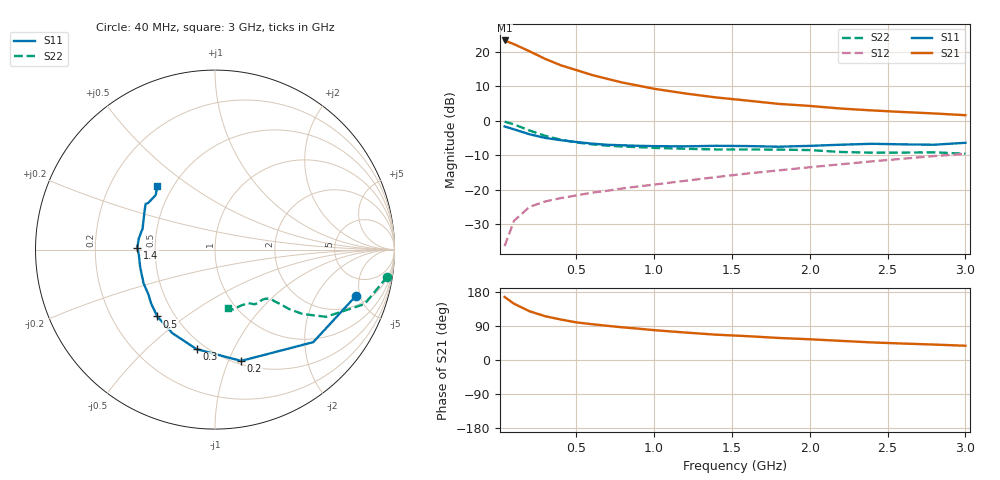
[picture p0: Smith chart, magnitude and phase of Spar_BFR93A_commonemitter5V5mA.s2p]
! Filename:  BFR93AA.S2P  Version:  2.0
! NXP part #: BFR93A  Date: May 1990
! Bias condition: Vce=5V, Ic=5mA
#  MHz  S  MA  R  50
! Freq  S11  S21  S12  S22  !GUM [dB]
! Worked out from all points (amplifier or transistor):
!   21 points, 40 MHz to 3 GHz, reference 50 ohm
!   highest |S21| = 23.4 dB at 40 MHz (marker M1)
!   |S21| within 3 dB of that: start of sweep to 192.8 MHz
!   unconditionally stable (mu >= 1): 1.032 GHz to 2.386 GHz
!   at 300 MHz: K = 0.48, MSG = 20.8 dB, |S12| = -23.5 dB
!   at 1 GHz: K = 0.99, MSG = 13.9 dB, |S12| = -18.6 dB
!   at 3 GHz: K = 0.95, MSG = 5.6 dB, |S12| = -9.6 dB
!   S11 on the Smith chart (normalised r, x): 40 MHz: 2.83, -4.60; 200 MHz: 0.53, -1.11; 300 MHz: 0.45, -0.73; 500 MHz: 0.40, -0.40; 1.4 GHz: 0.40, +0.01; 3 GHz: 0.41, +0.38
40  0.827 -18.1  14.76 166.3  0.015 78.6  0.972 -8.9
100  0.752 -43.3  13.04 148.6  0.035 68.3  0.887 -20.0
200  0.637 -76.8  10.27 128.6  0.056 56.9  0.723 -31.2
300  0.564 -100.5  7.982 115.6  0.067 52.2  0.606 -36.3
400  0.523 -116.9  6.438 106.9  0.075 51.1  0.531 -38.7
500  0.492 -130.8  5.481 99.4  0.082 51.3  0.485 -39.6
600  0.466 -139.7  4.652 94.5  0.09 52.2  0.455 -40.4
700  0.448 -145.7  4.077 90.2  0.096 54.3  0.435 -41.1
800  0.44 -154.6  3.59 86.1  0.104 56.1  0.422 -41.3
900  0.433 -159.7  3.245 82.6  0.111 58.0  0.414 -41.9
1000  0.428 -167.3  2.927 78.8  0.118 59.3  0.404 -42.5
1200  0.425 -175.6  2.5 72.5  0.134 61.9  0.392 -44.4
1400  0.433 178.5  2.186 66.8  0.152 64.0  0.383 -47.1
1600  0.429 171.6  1.968 62.9  0.171 65.9  0.383 -49.5
1800  0.42 163.9  1.763 58.2  0.19 66.4  0.381 -51.9
2000  0.432 157.0  1.647 54.7  0.211 67.4  0.375 -54.3
2200  0.449 150.8  1.508 50.5  0.233 68.5  0.352 -57.9
2400  0.463 146.6  1.417 46.4  0.257 67.8  0.344 -64.3
2600  0.454 145.2  1.342 43.4  0.281 67.6  0.345 -69.7
2800  0.449 137.3  1.279 40.7  0.307 67.0  0.348 -73.8
3000  0.479 132.2  1.207 37.6  0.331 65.8  0.332 -77.2
